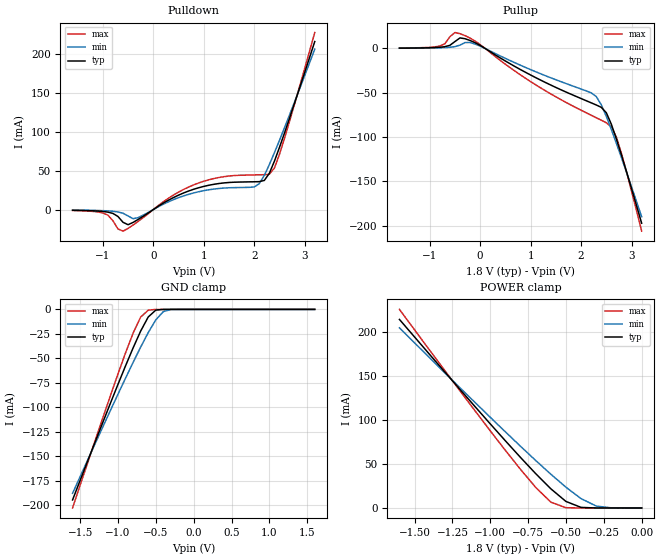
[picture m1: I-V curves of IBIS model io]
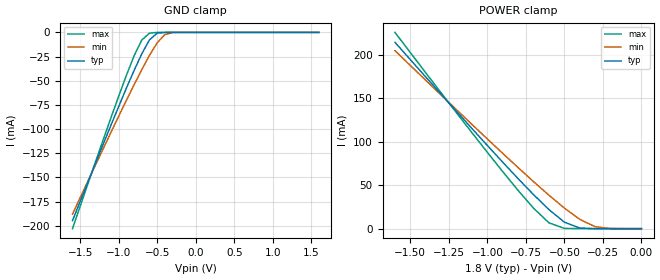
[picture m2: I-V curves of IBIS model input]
[IBIS Ver]	2.1
[File Name]	69r736c.ibs
[File Rev]	1.1
[Date]	8/31/99
[Source]	File originated at Motorola
[Notes]	This file is valid for:  MCM69R736C
|		(the 4M Late Write HSTL FSRAM).
|		BEWARE! This model has been generated with the
|		HSTL programmed to 50 impedance. The HSTL is capable
|		of impedances from 35ohms to 70 ohms.  This device is
|		internally regulated.  Model assumes a vddq = 1.5V
|		and a vref = 0.75V.
[Disclaimer]This information is for modeling purposes only and
|		is not guaranteed.
[Component]		128Kx36FSRAM
[Manufacturer]	Motorola
[Package]
|  RLC Data is subject to change after further study of package
|		typ		min		max
R_pkg		100m		NA		NA
L_pkg		5nH		NA		NA
C_pkg		1.5pF		NA		NA
[Pin]		signal_name	model_name	R_pin		L_pin		C_pin
1A		VDDQ		POWER		NA		NA		NA
1B		NC		NC		NA		NA		NA
1C		NC		NC		NA		NA		NA
1D		DQc		io		NA		NA		NA
1E		DQc		io		NA		NA		NA
1F		VDDQ		POWER		NA		NA		NA
1G		DQc		io		NA		NA		NA
1H		DQc		io		NA		NA		NA
1J		VDDQ		POWER		NA		NA		NA
1K		DQd		io		NA		NA		NA
1L		DQd		io		NA		NA		NA
1M		VDDQ		POWER		NA		NA		NA
1N		DQd		io		NA		NA		NA
1P		DQd		io		NA		NA		NA
1R		NC		NC		NA		NA		NA
1T		NC		NC		NA		NA		NA
1U		VDDQ		POWER		NA		NA		NA
2A		SA		input		NA		NA		NA
2B		NC	 	NC		NA		NA		NA
2C		SA		input		NA		NA		NA
2D		DQc		io		NA		NA		NA
2E		DQc		io		NA		NA		NA
2F		DQc		io		NA		NA		NA
2G		DQc		io		NA		NA		NA
2H		DQc		io		NA		NA		NA
2J		VDD		POWER		NA		NA		NA
2K		DQd		io		NA		NA		NA
2L		DQd		io		NA		NA		NA
2M		DQd		io		NA		NA		NA
2N		DQd		io		NA		NA		NA
2P		DQd		io		NA		NA		NA
2R		SA		input		NA		NA		NA
2T		NC		NC		NA		NA		NA
2U		TMS		input		NA		NA		NA
3A		SA		input		NA		NA		NA
3B		SA		input		NA		NA		NA
3C		SA		input		NA		NA		NA
3D		VSS		GND		NA		NA		NA
3E		VSS		GND		NA		NA		NA
3F		VSS		GND		NA		NA		NA
3G		SBc#		input		NA		NA		NA
3H		VSS		GND		NA		NA		NA
3J		Vref		POWER		NA		NA		NA
3K		VSS		GND		NA		NA		NA
3L		SBd#		input		NA		NA		NA
3M		VSS		GND		NA		NA		NA
3N		VSS		GND		NA		NA		NA
3P		VSS		GND		NA		NA		NA
3R		VSS		GND		NA		NA		NA
3T		SA		input		NA		NA		NA
3U		TDI		input		NA		NA		NA
4A		NC		NC		NA		NA		NA
4B		NC		NC		NA		NA		NA
4C		VDD		POWER		NA		NA		NA
4D		ZQ		NC		NA		NA		NA
4E		SS#		input		NA		NA		NA
4F		G#		input		NA		NA		NA
4G		NC		NC		NA		NA		NA
4H		NC		NC		NA		NA		NA
4J		VDD		POWER		NA		NA		NA
4K		CK		input		NA		NA		NA
4L		CK#		input		NA		NA		NA
4M		SW#		input		NA		NA		NA
4N		SA		input		NA		NA		NA
4P		SA		input		NA		NA		NA
4R		VDD		POWER		NA		NA		NA
4T		SA		input		NA		NA		NA
4U		TCK		input		NA		NA		NA
5A		SA		input		NA		NA		NA
5B		SA		input		NA		NA		NA
5C		SA		input		NA		NA		NA
5D		VSS		GND		NA		NA		NA
5E		VSS		GND		NA		NA		NA
5F		VSS		GND		NA		NA		NA
5G		SBb#		input		NA		NA		NA
5H		VSS		GND		NA		NA		NA
5J		Vref		POWER		NA		NA		NA
5K		VSS		GND		NA		NA		NA
5L		SBa#		input		NA		NA		NA
5M		VSS		GND		NA		NA		NA
5N		VSS		GND		NA		NA		NA
5P		VSS		GND		NA		NA		NA
5R		VDD		POWER		NA		NA		NA
5T		SA		input		NA		NA		NA
5U		TDO		input		NA		NA		NA
6A		SA		input		NA		NA		NA
6B		NC		NC		NA		NA		NA
6C		SA		input		NA		NA		NA
6D		DQb		io		NA		NA		NA
6E		DQb		io		NA		NA		NA
6F		DQb		io		NA		NA		NA
6G		DQb		io		NA		NA		NA
6H		DQb		io		NA		NA		NA
6J		VDD		POWER		NA		NA		NA
6K		DQa		io		NA		NA		NA
6L		DQa		io		NA		NA		NA
6M		DQa		io		NA		NA		NA
6N		DQa		io		NA		NA		NA
6P		DQa		io		NA		NA		NA
6R		SA		input		NA		NA		NA
6T		NC		NC		NA		NA		NA
6U		NC		NC		NA		NA		NA
7A		VDDQ		POWER		NA		NA		NA
7B		NC		NC		NA		NA		NA
7C		NC		NC		NA		NA		NA
7D		DQb		io		NA		NA		NA
7E		DQb		io		NA		NA		NA
7F		VDDQ		POWER		NA		NA		NA
7G		DQb		io		NA		NA		NA
7H		DQb		io		NA		NA		NA
7J		VDDQ		POWER		NA		NA		NA
7K		DQa		io		NA		NA		NA
7L		DQa		io		NA		NA		NA
7M		VDDQ		POWER		NA		NA		NA
7N		DQa		io		NA		NA		NA
7P		DQa		io		NA		NA		NA
7R		NC		NC		NA		NA		NA
7T		NC		NC		NA		NA		NA
7U		VDDQ		POWER		NA		NA		NA
| Models and submodels in the file (2): io (I/O), input (Input)
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[Model]	io
Model_type	I/O
Polarity	Non-Inverting
Enable	Active-Low
|		signals  DQa, DQb, DQc, DQd
|		typ		min		max
C_comp	6pF		5pF		8pF
|   |   |\ |   Rref
|   |Driver| \|------o----/\/\/\----o Vref
|   |   | /|   |
|   |   |/ |   === Cref
|   GND
Cref = 20pF
Rref = 50
Vref = 0.75
Vmeas = 0.75
Vinl = 0.55
Vinh = 0.95
|			typ		min		max
[Voltage range]	1.8V		1.6V		2.0V
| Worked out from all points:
|   slope of the pulldown table from 0 to 0.27 V, typ, clamps not added: 24.7 ohm
|   slope of the pullup table from 0 to 0.27 V, typ, clamps not added: 27.9 ohm
|   GND clamp passes 1 mA (typ) near -0.50 V on its own axis
|   POWER clamp passes 1 mA (typ) near -0.40 V on its own axis
| Temperature   50 C		110 C		0 C
[Pullup]
|	Voltage  	I(typ)   I(min)   I(max)
-1.6V     374.5uA    271.6uA    503uA
-800mV    1.401mA    770.5uA    2.752mA
-500mV    7.852mA    2.089mA    18.03mA
-400mV    11.93mA    3.813mA    16.71mA
-100mV    6.513mA    5.001mA    8.376mA
1V        -29.94mA   -23.86mA   -37.38mA
2.2V      -61.33mA   -50.07mA   -75.35mA
2.3V      -63.74mA   -54.19mA   -78.16mA
2.5V      -72.52mA   -76.67mA   -83.83mA
2.6V      -85.54mA   -91.51mA   -88.44mA
2.7V      -102.2mA   -107.2mA   -100.2mA
3.2V      -197.2mA   -189.9mA   -206.1mA
[Pulldown]
|	Voltage  	I(typ)   I(min)   I(max)
-1.6V     -920uA     -663uA     -1.209mA
-1V       -2.423mA   -1.404mA   -4.349mA
-800mV    -4.961mA   -2.211mA   -14.38mA
-600mV    -16.34mA   -4.739mA   -27.67mA
-300mV    -12.65mA   -10.37mA   -15.19mA
800mV     26.05mA    21.35mA    31.7mA
2V        35.69mA    29.04mA    44.49mA
2.2V      37.37mA    43.89mA    44.78mA
2.3V      46.6mA     57.75mA    45.38mA
2.4V      62.05mA    72.94mA    53.29mA
2.5V      79.68mA    88.79mA    70.83mA
3.2V      215.7mA    205.9mA    227.3mA
|   TRI-STATED OUTPUT
|   typ		min		max
|Voltage range	1.8V		1.6V		2.0V
| Temperature   50 C		110 C		0 C
|****************  FOR OUTPUTS  *********
[GND_clamp]
|	Voltage  	I(typ)   I(min)   I(max)
-1.6V     -194.7mA   -188mA     -203mA
-1.2V     -115.4mA   -120.1mA   -110.8mA
-900mV    -57.7mA    -70.28mA   -44.43mA
-800mV    -39.35mA   -54.16mA   -24.25mA
-700mV    -22.13mA   -38.51mA   -7.832mA
-600mV    -7.722mA   -23.7mA    -807.3uA
-500mV    -739.8uA   -10.7mA    -22.45uA
-400mV    -25.95uA   -2.225mA   -727.9nA
-300mV    -895.2nA   -154.9uA   -24.79nA
1.6V      509.5pA    366.3nA    43.35pA
[POWER_clamp]
|	Voltage  	I(typ)   I(min)   I(max)
-1.6V     214.7mA    205.1mA    226.1mA
-1.2V     135mA      136.9mA    133.4mA
-900mV    76.47mA    86.66mA    65.57mA
-700mV    39.13mA    54.12mA    23.5mA
-600mV    21.88mA    38.48mA    6.666mA
-500mV    7.459mA    23.67mA    295.1uA
-400mV    671.7uA    10.67mA    4.439uA
-300mV    20.74uA    2.208mA    63.53nA
-200mV    573.9nA    152uA      960.3pA
0V        509.5pA    366.3nA    43.35pA
[Ramp]
| 		typ			min			max
|Temperature  50 C		110 C			0 C
dV/dt_r	0.385/0.089n	0.314/0.095n	0.429/0.072n
dV/dt_f	0.397/0.111n	0.342/0.129n	0.494/0.114n
[Model]		input
Model_type		Input
Polarity		Non-Inverting
| signals  SA, G#,  SS#, SBa#, SBb#, SBc#, SBd#, CK#, CK,
|   TDI,  TMS,  TCK, SW#, ZQ, TDO
|  	* TDO has been listed here, but it is technically an output pin.
| 	This simplification has been made under the assumption
|  	that its structure is similar to the input pin's structure.
Vinl = 0.65V
Vinh = 0.85V
|			typ		min		max
C_comp		5pF		4pF		5pF
|			typ		min		max
[Voltage range]	1.8V		1.6V		2.0V
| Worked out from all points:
|   GND clamp passes 1 mA (typ) near -0.50 V on its own axis
|   POWER clamp passes 1 mA (typ) near -0.40 V on its own axis
| Temperature   50 C		110 C		0 C
[GND_clamp]
|	Voltage  	I(typ)   I(min)   I(max)
-1.6V     -194.7mA   -188mA     -203mA
-1.2V     -115.4mA   -120.1mA   -110.8mA
-900mV    -57.7mA    -70.28mA   -44.43mA
-800mV    -39.35mA   -54.16mA   -24.25mA
-700mV    -22.13mA   -38.51mA   -7.832mA
-600mV    -7.722mA   -23.7mA    -807.3uA
-500mV    -739.8uA   -10.7mA    -22.45uA
-400mV    -25.95uA   -2.225mA   -727.9nA
-300mV    -895.2nA   -154.9uA   -24.79nA
1.6V      509.5pA    366.3nA    43.35pA
[POWER_clamp]
|	Voltage	I(typ)		I(min)		I(max)
-1.6V     214.7mA    205.1mA    226.1mA
-1.2V     135mA      136.9mA    133.4mA
-900mV    76.47mA    86.66mA    65.57mA
-700mV    39.13mA    54.12mA    23.5mA
-600mV    21.88mA    38.48mA    6.666mA
-500mV    7.459mA    23.67mA    295.1uA
-400mV    671.7uA    10.67mA    4.439uA
-300mV    20.74uA    2.208mA    63.53nA
-200mV    573.9nA    152uA      960.3pA
0V        509.5pA    366.3nA    43.35pA
